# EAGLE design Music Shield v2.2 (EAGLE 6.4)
music shield
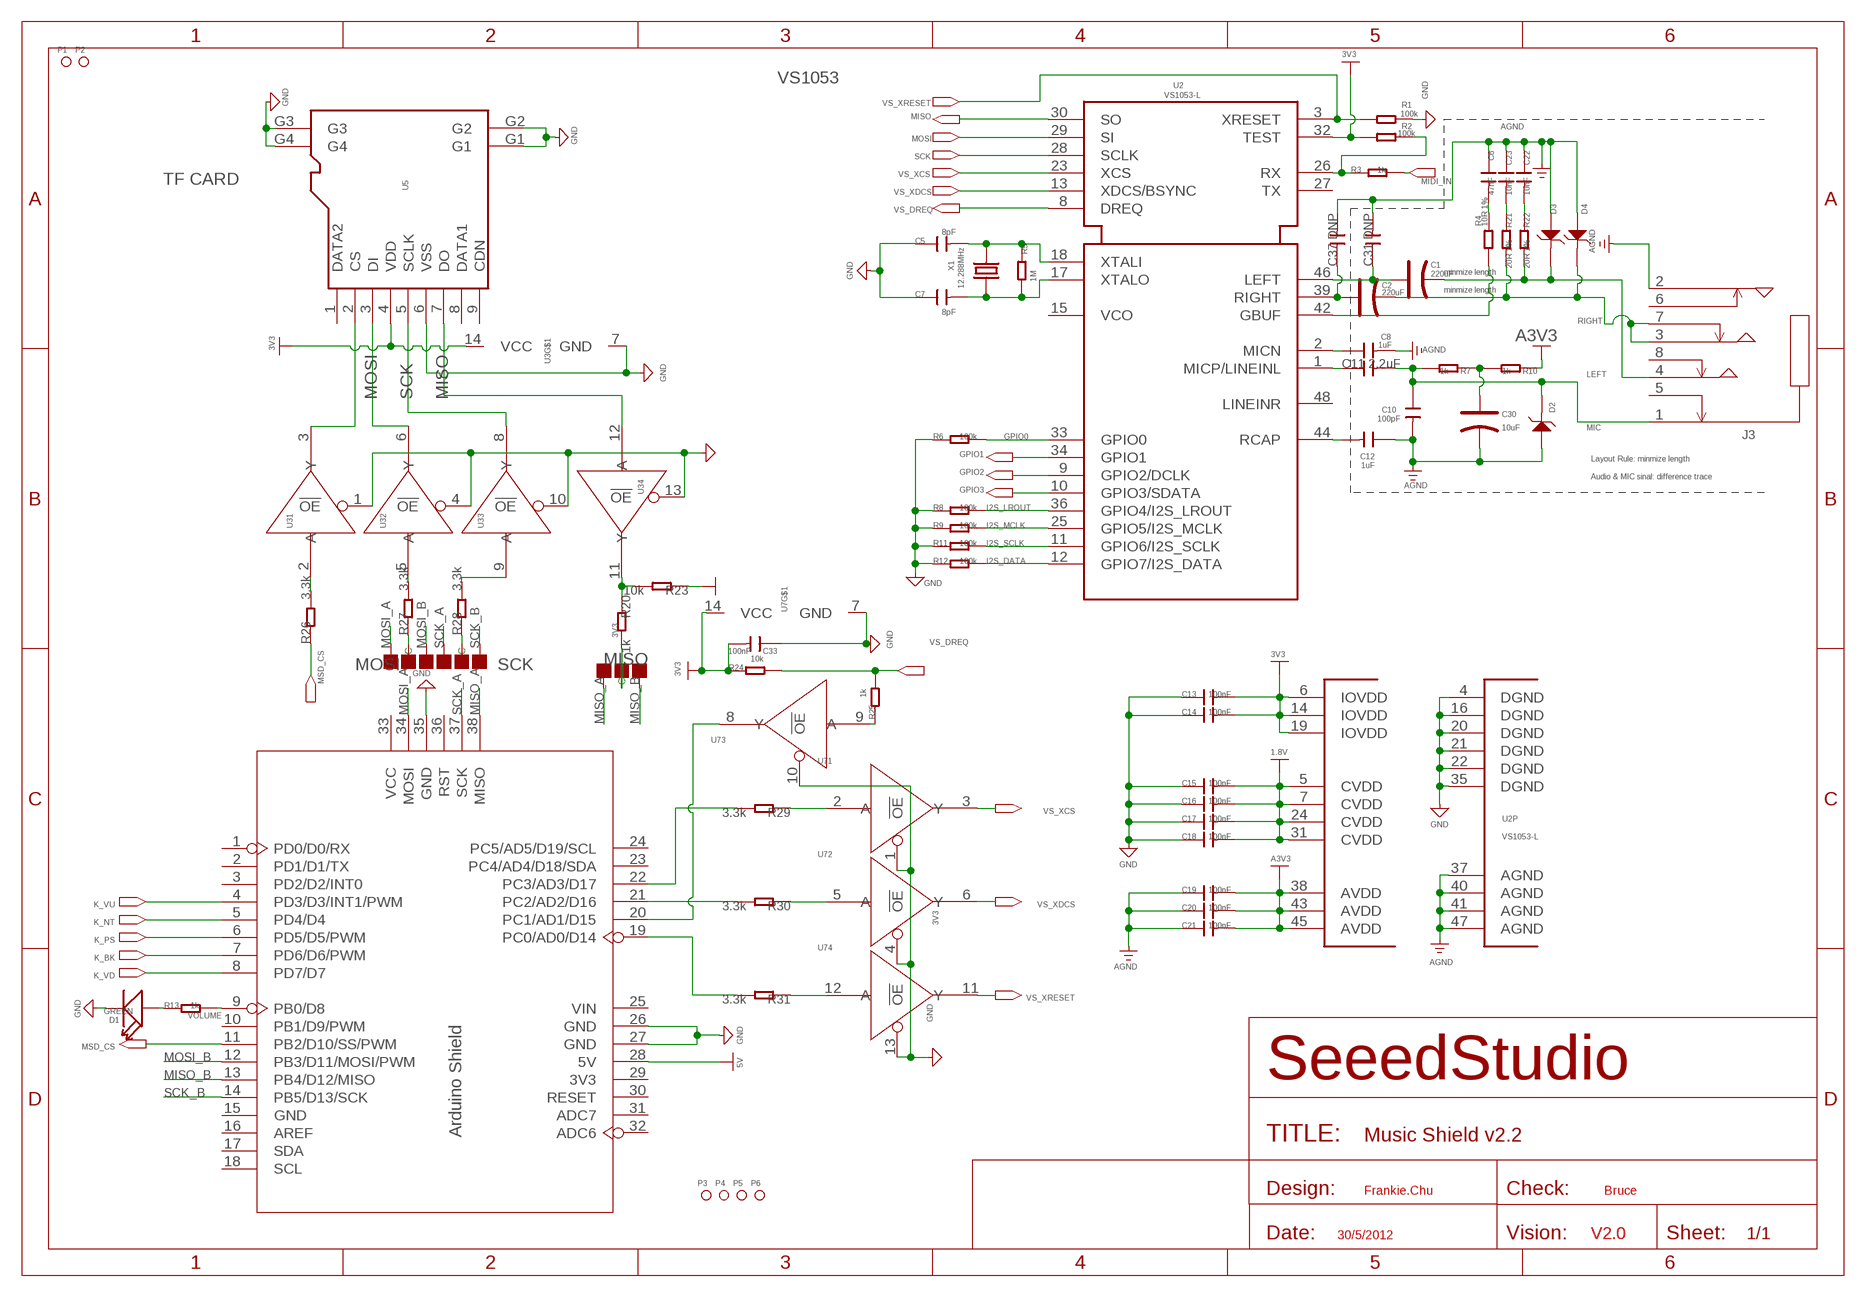
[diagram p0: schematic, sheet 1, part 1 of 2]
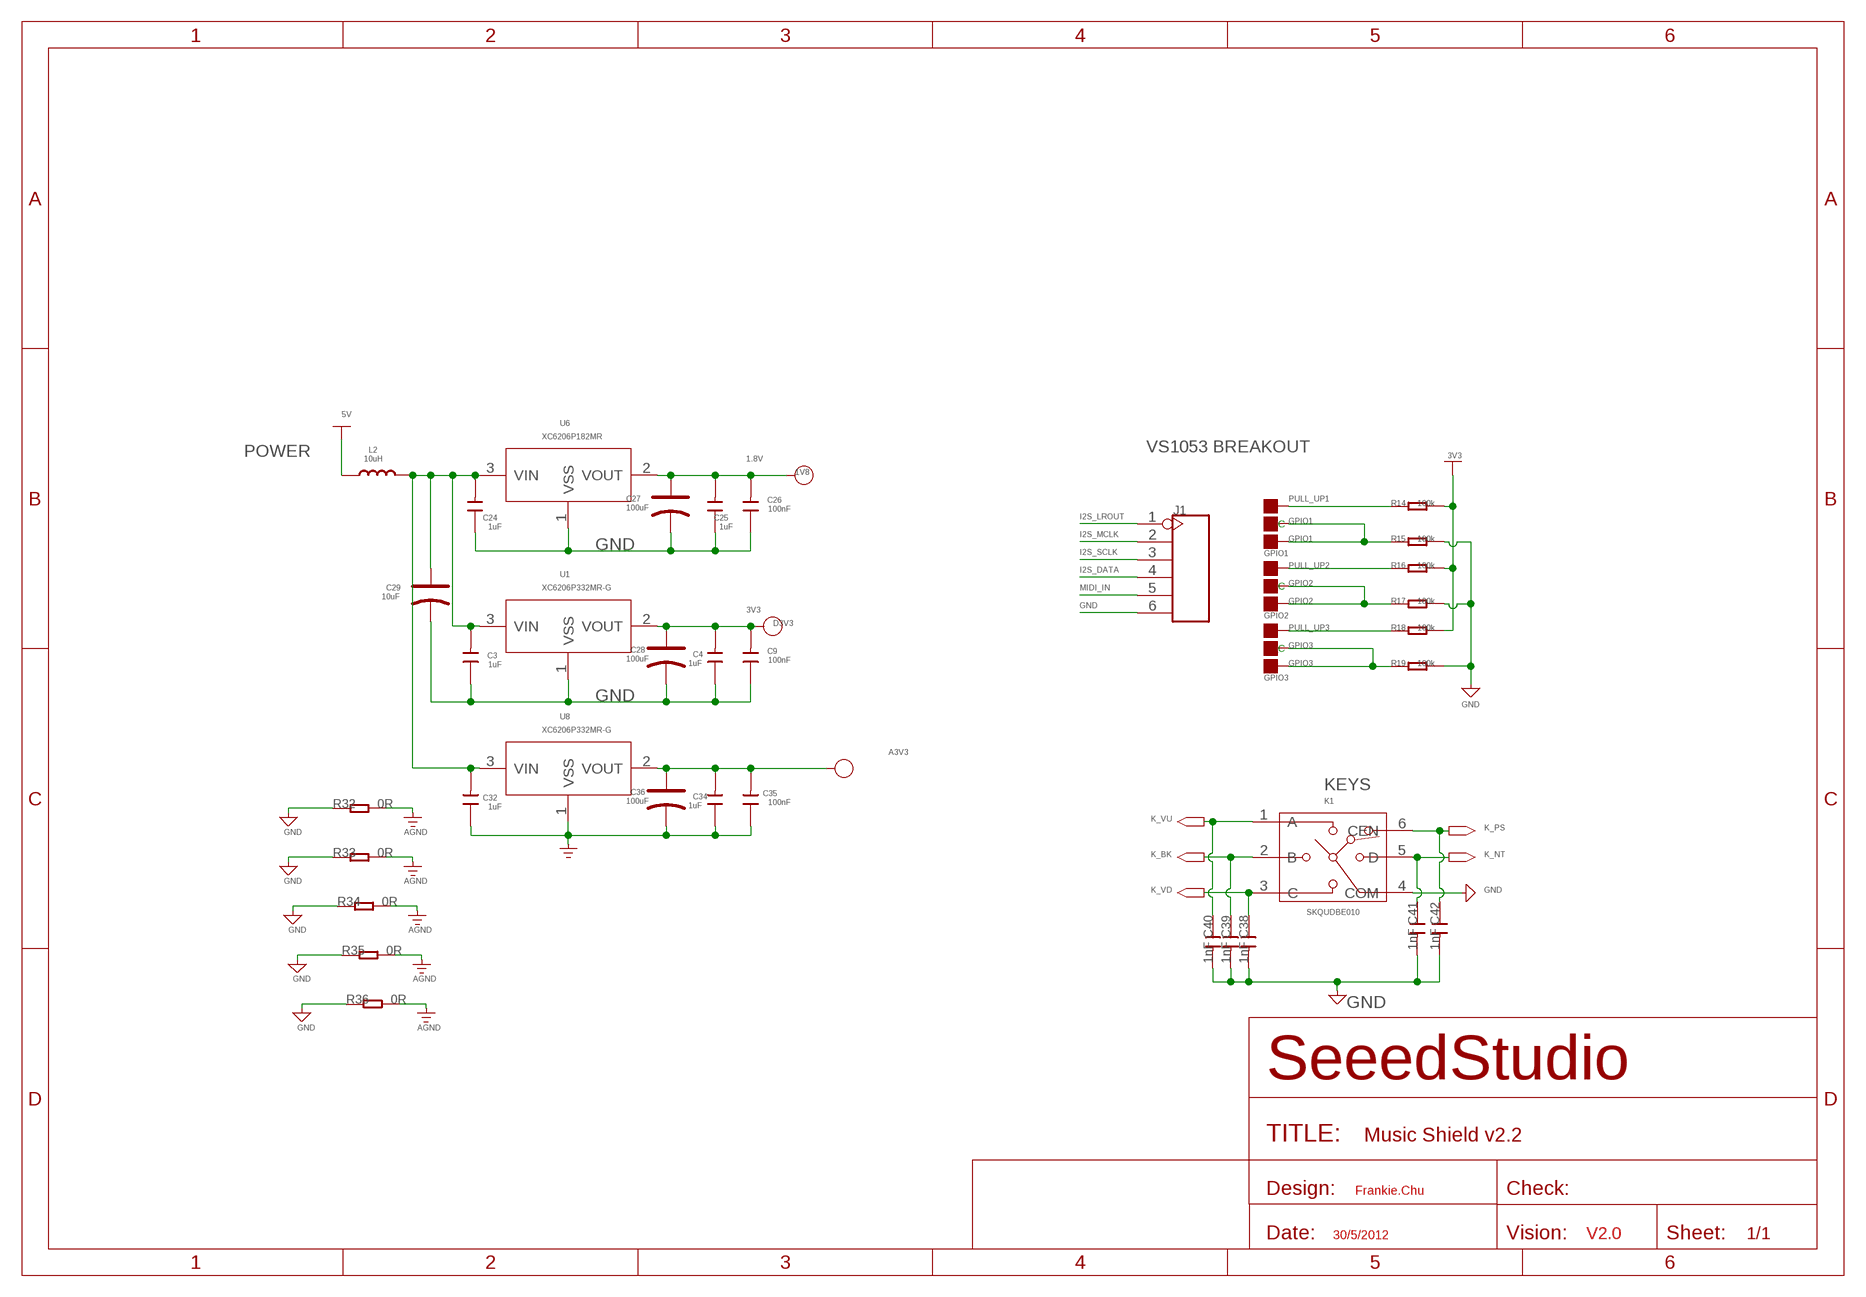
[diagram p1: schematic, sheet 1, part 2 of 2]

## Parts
1V8  PAD-TEST-POINT'4545'  [TP_4545]
A3V3  PAD-TEST-POINT'4545'  [TP_4545]
C1  220uF  CAP-AVX-B  [AVX-B]
C2  220uF  CAP-AVX-B  [AVX-B]
C3  1uF  C-0603  [C0603]
C4  1uF  C-0603  [C0603]
C5  8pF  C-0603  [C0603]
C6  47nF  C-0603  [C0603]
C7  8pF  C-0603  [C0603]
C8  1uF  C-0603  [C0603]
C9  100nF  C-0603  [C0603]
C10  100pF  C-0603  [C0603]
C11  2.2uF  C-0805  [C0805]
C12  1uF  C-0603  [C0603]
C13  100nF  C-0603  [C0603]
C14  100nF  C-0603  [C0603]
C15  100nF  C-0603  [C0603]
C16  100nF  C-0603  [C0603]
C17  100nF  C-0603  [C0603]
C18  100nF  C-0603  [C0603]
C19  100nF  C-0603  [C0603]
C20  100nF  C-0603  [C0603]
C21  100nF  C-0603  [C0603]
C22  10nF  C-0603  [C0603]
C23  10nF  C-0603  [C0603]
C24  1uF  C-0603  [C0603]
C25  1uF  C-0603  [C0603]
C26  100nF  C-0603  [C0603]
C27  100uF  CAP-AVX-B  [AVX-B]
C28  100uF  CAP-AVX-B  [AVX-B]
C29  10uF  CAP-AVX-A  [AVX-A]
C30  10uF  CAP-AVX-A  [AVX-A]
C31  DNP  C-0603  [C0603]
C32  1uF  C-0603  [C0603]
C33  100nF  C-0603  [C0603]
C34  1uF  C-0603  [C0603]
C35  100nF  C-0603  [C0603]
C36  100uF  CAP-AVX-B  [AVX-B]
C37  DNP  C-0603  [C0603]
C38  1nF  C-0603  [C0603]
C39  1nF  C-0603  [C0603]
C40  1nF  C-0603  [C0603]
C41  1nF  C-0603  [C0603]
C42  1nF  C-0603  [C0603]
D1  GREEN  LED'0603'  [LED-0603]
D2  CESD5V0D1  D-ESD  [SOD123-2.7X1.6]
D3  CESD5V0D1  D-ESD  [SOD123-2.7X1.6]
D3V3  PAD-TEST-POINT'4545'  [TP_4545]
D4  CESD5V0D1  D-ESD  [SOD123-2.7X1.6]
GPIO1  PAD-JUMPER-3P-40*40  [3P-SMD-4.1X1.5]
GPIO2  PAD-JUMPER-3P-40*40  [3P-SMD-4.1X1.5]
GPIO3  PAD-JUMPER-3P-40*40  [3P-SMD-4.1X1.5]
J1  HEADER-6P-55/35MIL  [6P-2.54-55/35MIL]
J3  AUDIO-JACK-3.5'PJ-393'  [8P-SMD-3.5]
K1  SKQUDBE010  [6P-10X10X8.6MM]
L2  10uH  L'0806'  [0806]
MISO  PAD-JUMPER-3P-40*40  [3P-SMD-4.1X1.5]
MOSI  PAD-JUMPER-3P-40*40  [3P-SMD-4.1X1.5]
P1  PAD-MARK'ANNULAR'  [ROUND-MARK-1.0]
P2  PAD-MARK'ANNULAR'  [ROUND-MARK-1.0]
P3  PAD-MARK'ANNULAR'  [ROUND-MARK-1.0]
P4  PAD-MARK'ANNULAR'  [ROUND-MARK-1.0]
P5  PAD-MARK'ANNULAR'  [ROUND-MARK-1.0]
P6  PAD-MARK'ANNULAR'  [ROUND-MARK-1.0]
R1  100k  R-0603  [R0603]
R2  100k  R-0603  [R0603]
R3  1k  R-0603  [R0603]
R4  10R 1%  R-0603  [R0603]
R5  1M  R-0603  [R0603]
R6  100k  R-0603  [R0603]
R7  1k  R-0603  [R0603]
R8  100k  R-0603  [R0603]
R9  100k  R-0603  [R0603]
R10  1k  R-0603  [R0603]
R11  100k  R-0603  [R0603]
R12  100k  R-0603  [R0603]
R13  1k  R-0603  [R0603]
R14  100k  R-0603  [R0603]
R15  100k  R-0603  [R0603]
R16  100k  R-0603  [R0603]
R17  100k  R-0603  [R0603]
R18  100k  R-0603  [R0603]
R19  100k  R-0603  [R0603]
R20  1k  R-0603  [R0603]
R21  20R 1%  R-0603  [R0603]
R22  20R 1%  R-0603  [R0603]
R23  10k  R-0603  [R0603]
R24  10k  R-0603  [R0603]
R25  1k  R-0603  [R0603]
R26  3.3k  R-0603  [R0603]
R27  3.3k  R-0603  [R0603]
R28  3.3k  R-0603  [R0603]
R29  3.3k  R-0603  [R0603]
R30  3.3k  R-0603  [R0603]
R31  3.3k  R-0603  [R0603]
R32  0R  R-0603  [R0603]
R33  0R  R-0603  [R0603]
R34  0R  R-0603  [R0603]
R35  0R  R-0603  [R0603]
R36  0R  R-0603  [R0603]
SCK  PAD-JUMPER-3P-40*40  [3P-SMD-4.1X1.5]
U1  XC6206P332MR-G  XC6206MR  [SOT23]
U2  VS1053-L  [LQFP48]
U3  74VHC125MTCX  74VHC125PW  [TSSOP14]
U5  HOLDER-MICROSD-9P'HOLDER'  [9P-SMD-W/-RING]
U6  XC6206P182MR  XC6206MR  [SOT23]
U7  74VHC125MTCX  74VHC125PW  [TSSOP14]
U8  XC6206P332MR-G  XC6206MR  [SOT23]
U10  ARDUINO-38P'WITH/O-SILK'  [ARDUINO-38P-500519002]
X1  12.288MHz  CRYSTAL'5032'  [2P-SMD-5X3.2]

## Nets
1.8V: 1V8.T C15.2 C16.2 C17.2 C18.2 C25.2 C26.2 C27.+ U2.5(CVDD) U2.7(CVDD) U2.24(CVDD) U2.31(CVDD) U6.2(VOUT) ; supply symbol labelled POWER_BAR
3V3: C4.2 C9.2 C13.2 C14.2 C28.+ C33.2 D3V3.T R2.1 R14.2 R16.2 R18.2 R23.1 R24.1 U1.2(VOUT) U2.6(IOVDD) U2.14(IOVDD) U2.19(IOVDD) U2.32(TEST) U3.14(VCC) U5.4(VDD) U7.14(VCC) ; supply symbol labelled POWER_BAR
5V: L2.1 U10.28(5V) ; supply symbol labelled POWER_BAR
A3V3: A3V3.T C19.2 C20.2 C21.2 C34.2 C35.2 C36.+ R10.1 U2.38(AVDD) U2.43(AVDD) U2.45(AVDD) U8.2(VOUT) ; supply symbol labelled POWER_BAR
AGND: C6.1 C8.2 C10.2 C12.1 C19.1 C20.1 C21.1 C22.1 C23.1 C30.- C31.2 C32.1 C34.1 C35.1 C36.- C37.2 D2.1 D3.1 D4.1 J3.2 R32.2 R33.2 R34.2 R35.2 R36.2 U2.37(AGND) U2.40(AGND) U2.41(AGND) U2.47(AGND) U8.1(VSS)
GND: C3.1 C4.1 C5.1 C7.1 C9.1 C13.1 C14.1 C15.1 C16.1 C17.1 C18.1 C24.1 C25.1 C26.1 C27.- C28.- C29.- C33.1 C38.2 C39.2 C40.2 C41.2 C42.2 D1.- J1.6 K1.4(COM) R1.2 R6.1 R8.1 R9.1 R11.1 R12.1 R15.2 R17.2 R19.2 R32.1 R33.1 R34.1 R35.1 R36.1 U1.1(VSS) U2.4(DGND) U2.16(DGND) U2.20(DGND) U2.21(DGND) U2.22(DGND) U2.35(DGND) U3.1(1:!OE) U3.4(2:!OE) U3.7(GND) U3.10(3:!OE) U3.13(4:!OE) U5.6(VSS) U5.G1 U5.G2 U5.G3 U5.G4 U6.1(VSS) U7.1(1:!OE) U7.4(2:!OE) U7.7(GND) U7.10(3:!OE) U7.13(4:!OE) U10.26(GND) U10.27(GND) U10.35(GND) ; supply symbol labelled GND_SIGNAL
GPIO0: R6.2 U2.33(GPIO0)
GPIO1: GPIO1.00(L) GPIO1.MM(C) R15.1 U2.34(GPIO1)
GPIO2: GPIO2.00(L) GPIO2.MM(C) R17.1 U2.9(GPIO2/DCLK)
GPIO3: GPIO3.00(L) GPIO3.MM(C) R19.1 U2.10(GPIO3/SDATA)
I2S_DATA: J1.4 R12.2 U2.12(GPIO7/I2S_DATA)
I2S_LROUT: J1.1 R8.2 U2.36(GPIO4/I2S_LROUT)
I2S_MCLK: J1.2 R9.2 U2.25(GPIO5/I2S_MCLK)
I2S_SCLK: J1.3 R11.2 U2.11(GPIO6/I2S_SCLK)
K_BK: C39.1 K1.2(B) U10.7(PD6/D6/PWM)
K_NT: C41.1 K1.5(D) U10.5(PD4/D4)
K_PS: C42.1 K1.6(CEN) U10.6(PD5/D5/PWM)
K_VD: C38.1 K1.3(C) U10.8(PD7/D7)
K_VU: C40.1 K1.1(A) U10.4(PD3/D3/INT1/PWM)
LEFT: C1.- D3.2 J3.4 R22.2
MIC: C10.1 C11.2 D2.2 J3.1 R7.2
MIDI_IN: J1.5 R3.2
MISO: U2.30(SO) U3.12(4:A) U5.7(DO)
MISO_A: MISO.00(L) U10.38(MISO)
MISO_B: MISO.11(R) U10.13(PB4/D12/MISO)
MOSI: U2.29(SI) U3.6(2:Y) U5.3(DI)
MOSI_A: MOSI.11(R) U10.34(MOSI)
MOSI_B: MOSI.00(L) U10.12(PB3/D11/MOSI/PWM)
MSD_CS: R26.1 U10.11(PB2/D10/SS/PWM)
N$1: C5.2 R5.1 U2.18(XTALI) X1.2
N$2: C7.2 R5.2 U2.17(XTALO) X1.1
N$3: C12.2 U2.44(RCAP)
N$4: C30.+ R7.1 R10.2
N$5: C22.2 R22.1
N$6: C2.+ C37.1 U2.39(RIGHT)
N$7: C8.1 U2.2(MICN)
N$8: C1.+ C31.1 U2.46(LEFT)
N$9: C6.2 R4.2
N$10: C23.2 R21.1
N$11: C11.1 U2.1(MICP/LINEINL)
N$12: R2.2 R3.1 U2.26(RX)
N$13: C3.2 C24.2 C29.+ C32.2 L2.2 U1.3(VIN) U6.3(VIN) U8.3(VIN)
N$14: R31.2 U10.19(PC0/AD0/D14)
N$15: R4.1 U2.42(GBUF)
N$16: R26.2 U3.2(1:A)
N$17: R29.1 U7.2(1:A)
N$18: R27.2 U3.5(2:A)
N$19: R30.1 U7.5(2:A)
N$20: R31.1 U7.12(4:A)
N$21: U3.3(1:Y) U5.2(CS)
N$22: R29.2 U10.22(PC3/AD3/D17)
N$23: R30.2 U10.21(PC2/AD2/D16)
N$24: U7.8(3:Y) U10.20(PC1/AD1/D15)
N$36: R20.1 R23.2 U3.11(4:Y)
N$37: D1.+ R13.1
N$38: R25.1 U7.9(3:A)
N$39: MISO.MM(C) R20.2
N$40: R28.2 U3.9(3:A)
N$49: MOSI.MM(C) R27.1
N$53: R28.1 SCK.MM(C)
PULL_UP1: GPIO1.11(R) R14.1
PULL_UP2: GPIO2.11(R) R16.1
PULL_UP3: GPIO3.11(R) R18.1
RIGHT: C2.- D4.2 J3.3 J3.7 R21.2
SCK: U2.28(SCLK) U3.8(3:Y) U5.5(SCLK)
SCK_A: SCK.11(R) U10.37(SCK)
SCK_B: SCK.00(L) U10.14(PB5/D13/SCK)
VOLUME: R13.2 U10.9(PB0/D8)
VS_DREQ: R24.2 R25.2 U2.8(DREQ)
VS_XCS: U2.23(XCS) U7.3(1:Y)
VS_XDCS: U2.13(XDCS/BSYNC) U7.6(2:Y)
VS_XRESET: R1.1 U2.3(XRESET) U7.11(4:Y)
Unconnected: J3.5 J3.6 J3.8 U2.15(VCO) U2.27(TX) U2.48(LINEINR) U5.1(DATA2) U5.8(DATA1) U5.9(CDN) U10.1(PD0/D0/RX) U10.2(PD1/D1/TX) U10.3(PD2/D2/INT0) U10.10(PB1/D9/PWM) U10.15(GND) U10.16(AREF) U10.17(SDA) U10.18(SCL) U10.23(PC4/AD4/D18/SDA) U10.24(PC5/AD5/D19/SCL) U10.25(VIN) U10.29(3V3) U10.30(RESET) U10.31(ADC7) U10.32(ADC6) U10.33(VCC) U10.36(RST)

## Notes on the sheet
- VS1053
- TF CARD
- minmize length
- minmize length
- POWER | VS1053 BREAKOUT
- Layout Rule: minmize length
- Audio & MIC sinal: difference trace
- KEYS
- Arduino Shield
- Frankie.Chu | Bruce | Frankie.Chu
- 30/5/2012 | V2.0 | 30/5/2012 | V2.0

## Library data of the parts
1V8 A3V3 D3V3 = Discrete:PAD-TEST-POINT; PARTNO: DNP
C1 C2 C27-C30 C36 = Discrete:CAP*: Electrolytic Capacitors,Tantalum Capacitors and Super Capacitors
C3-C26 C31-C35 C37-C42 = Discrete:C*: Ceramic Capacitors
D1 = Discrete:LED*
D2-D4 = template:D-ESD: Diodes for Protectiong against ESD
GPIO1-GPIO3 MISO MOSI SCK = Discrete:PAD-JUMPER-3P; PARTNO: DNP
J1 = Connector:HEADER-6P
J3 = template:AUDIO-JACK-3.5
K1 = template:SKQUDBE010: four dircction and center button
L2 = Discrete:L*
P1-P6 = Discrete:PAD-MARK; PARTNO: DNP
R1-R36 = Discrete:R*
U1 U6 U8 = IC:XC6206: LOW ESR Cap.Compatible Positive Voltage Regulators
U2 = vlsi:VS1053
U3 U7 = template:74V*125: Quad Buffer/Line Driver;3-state
U5 = Connector:HOLDER-MICROSD-9P
U10 = moudle:ARDUINO-38P
X1 = Discrete:CRYSTAL*: CRYSTAL

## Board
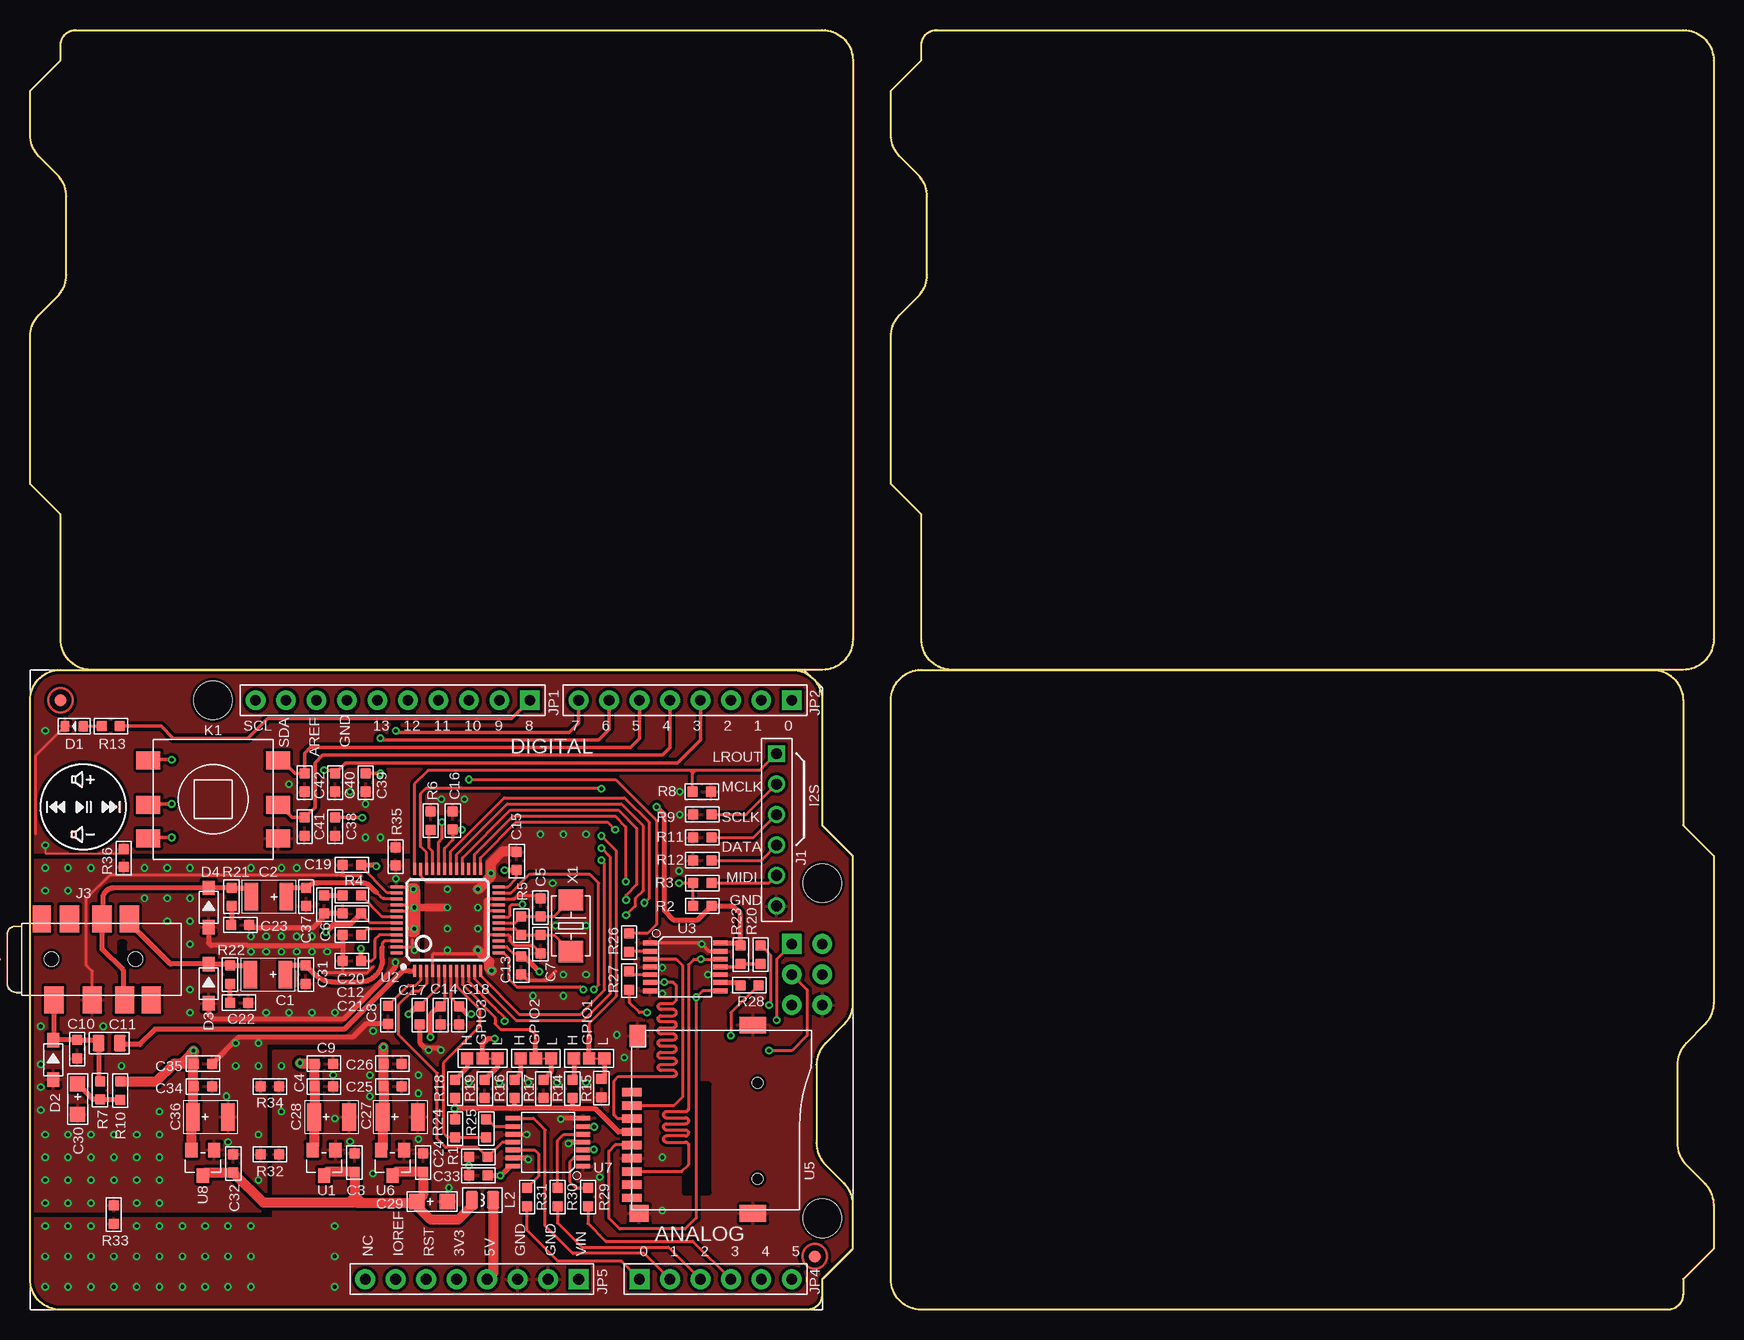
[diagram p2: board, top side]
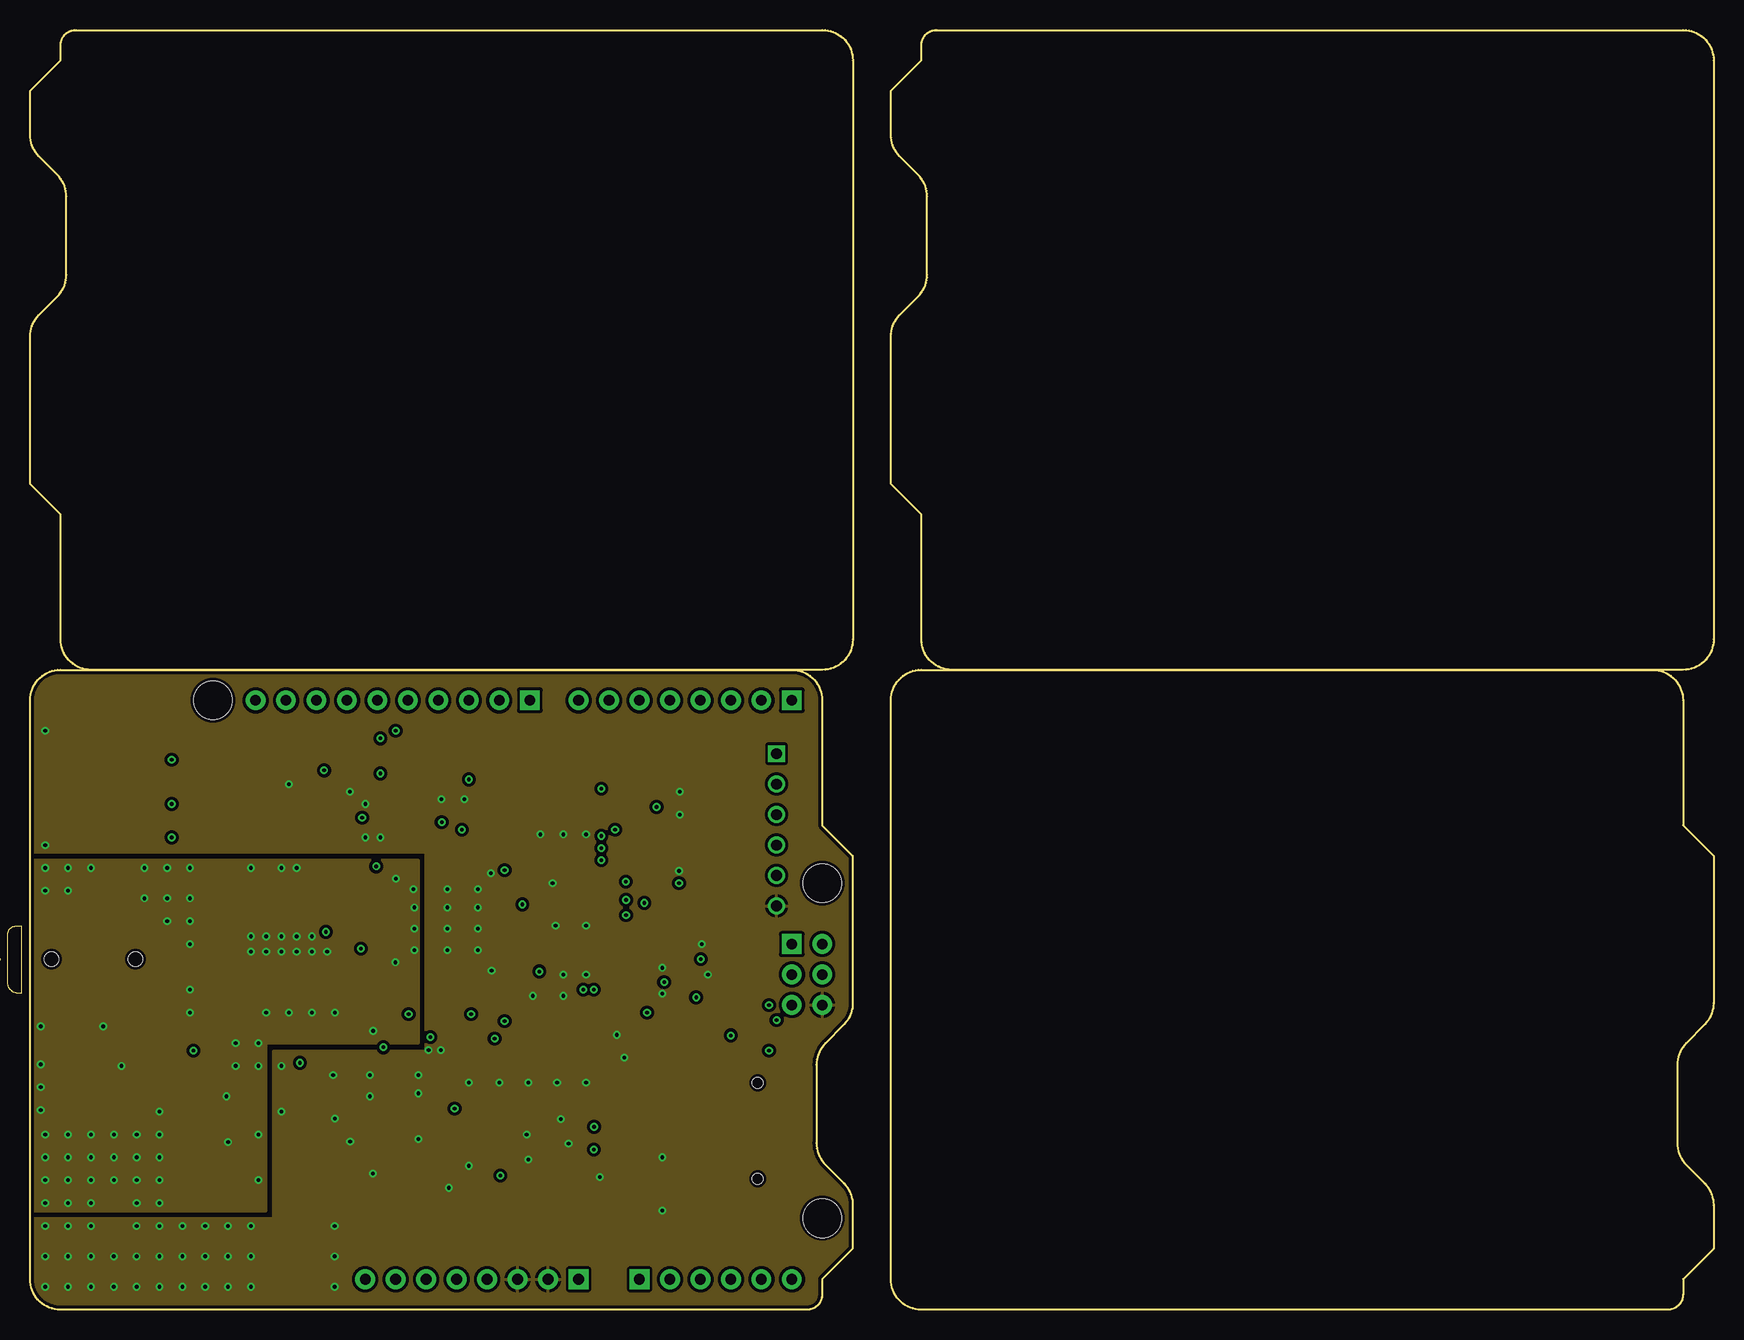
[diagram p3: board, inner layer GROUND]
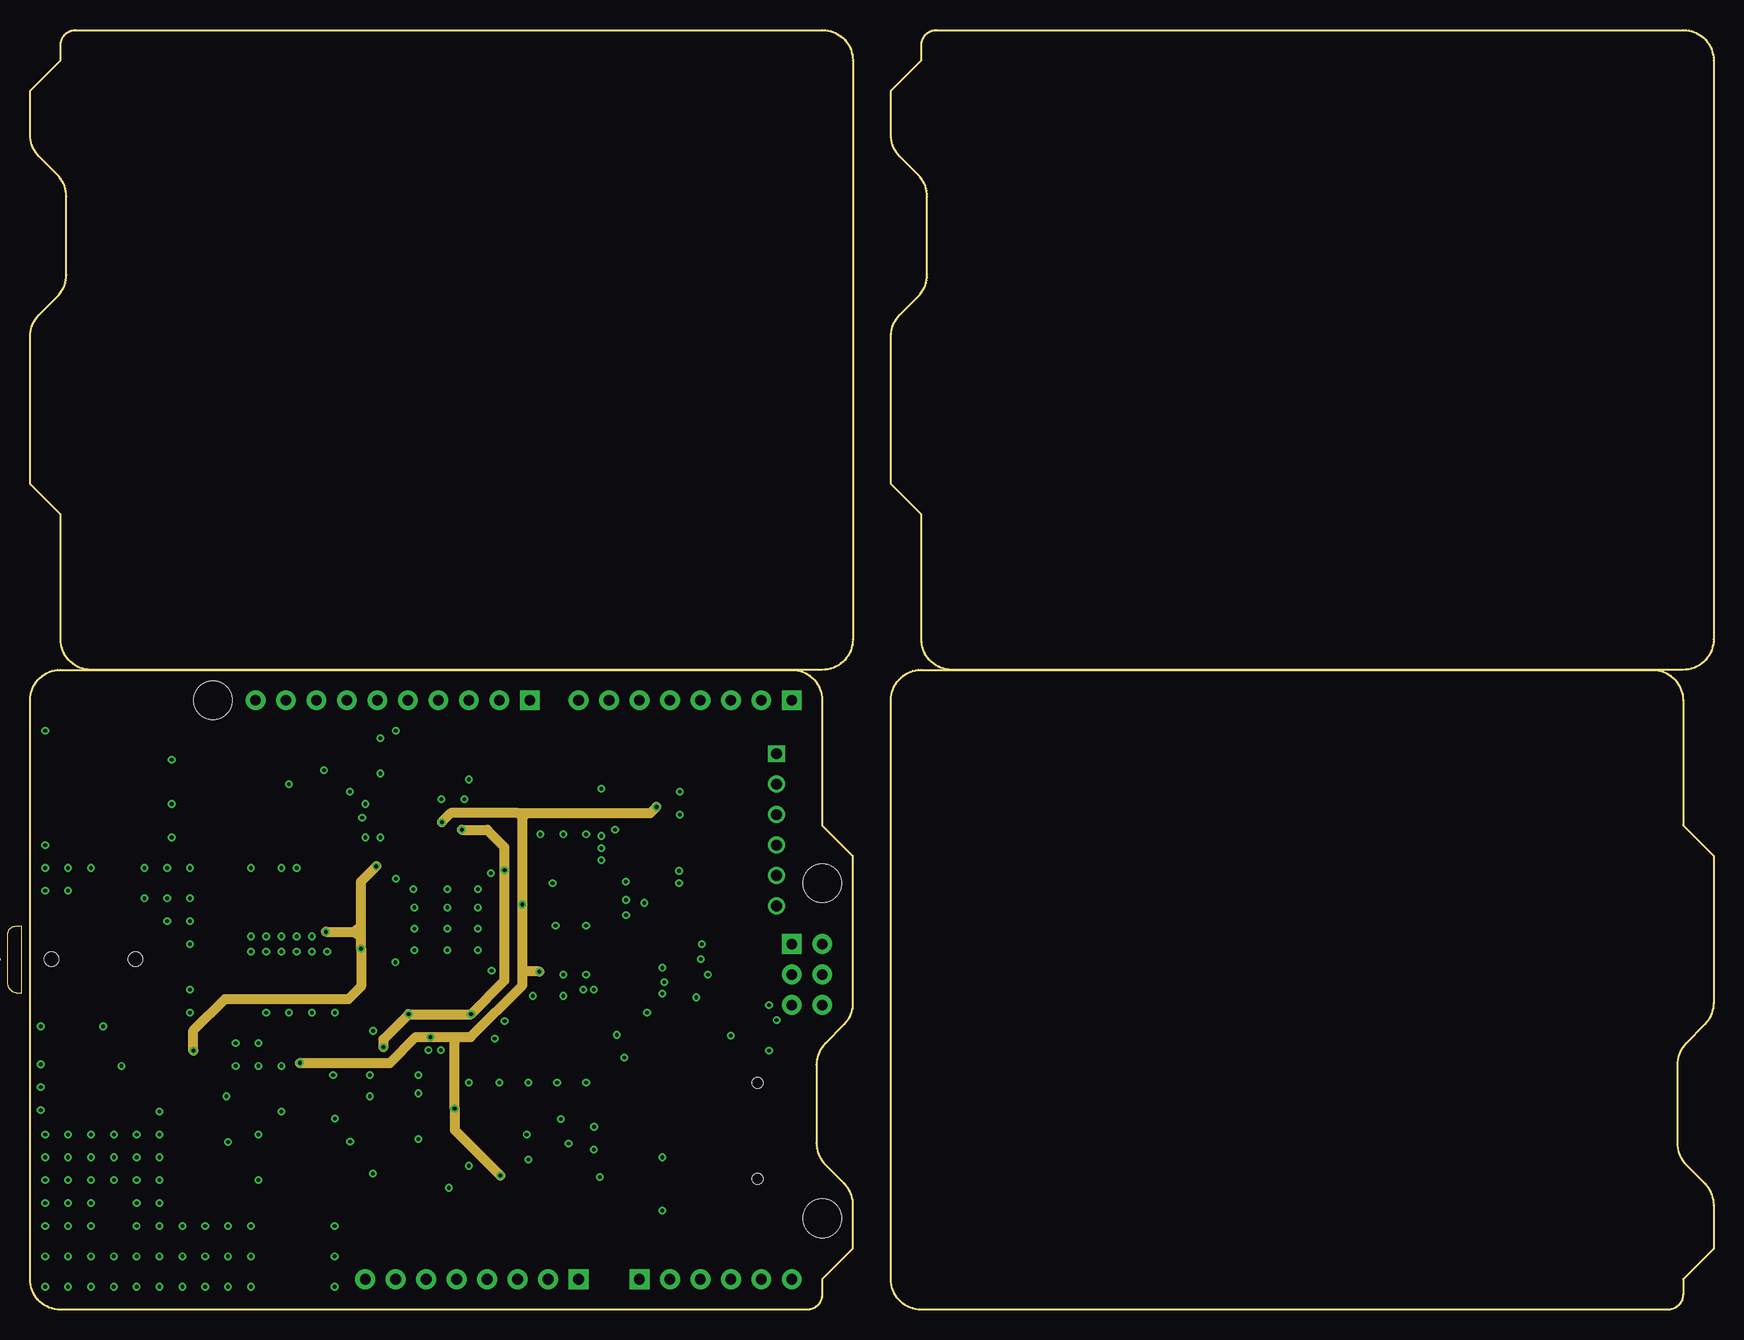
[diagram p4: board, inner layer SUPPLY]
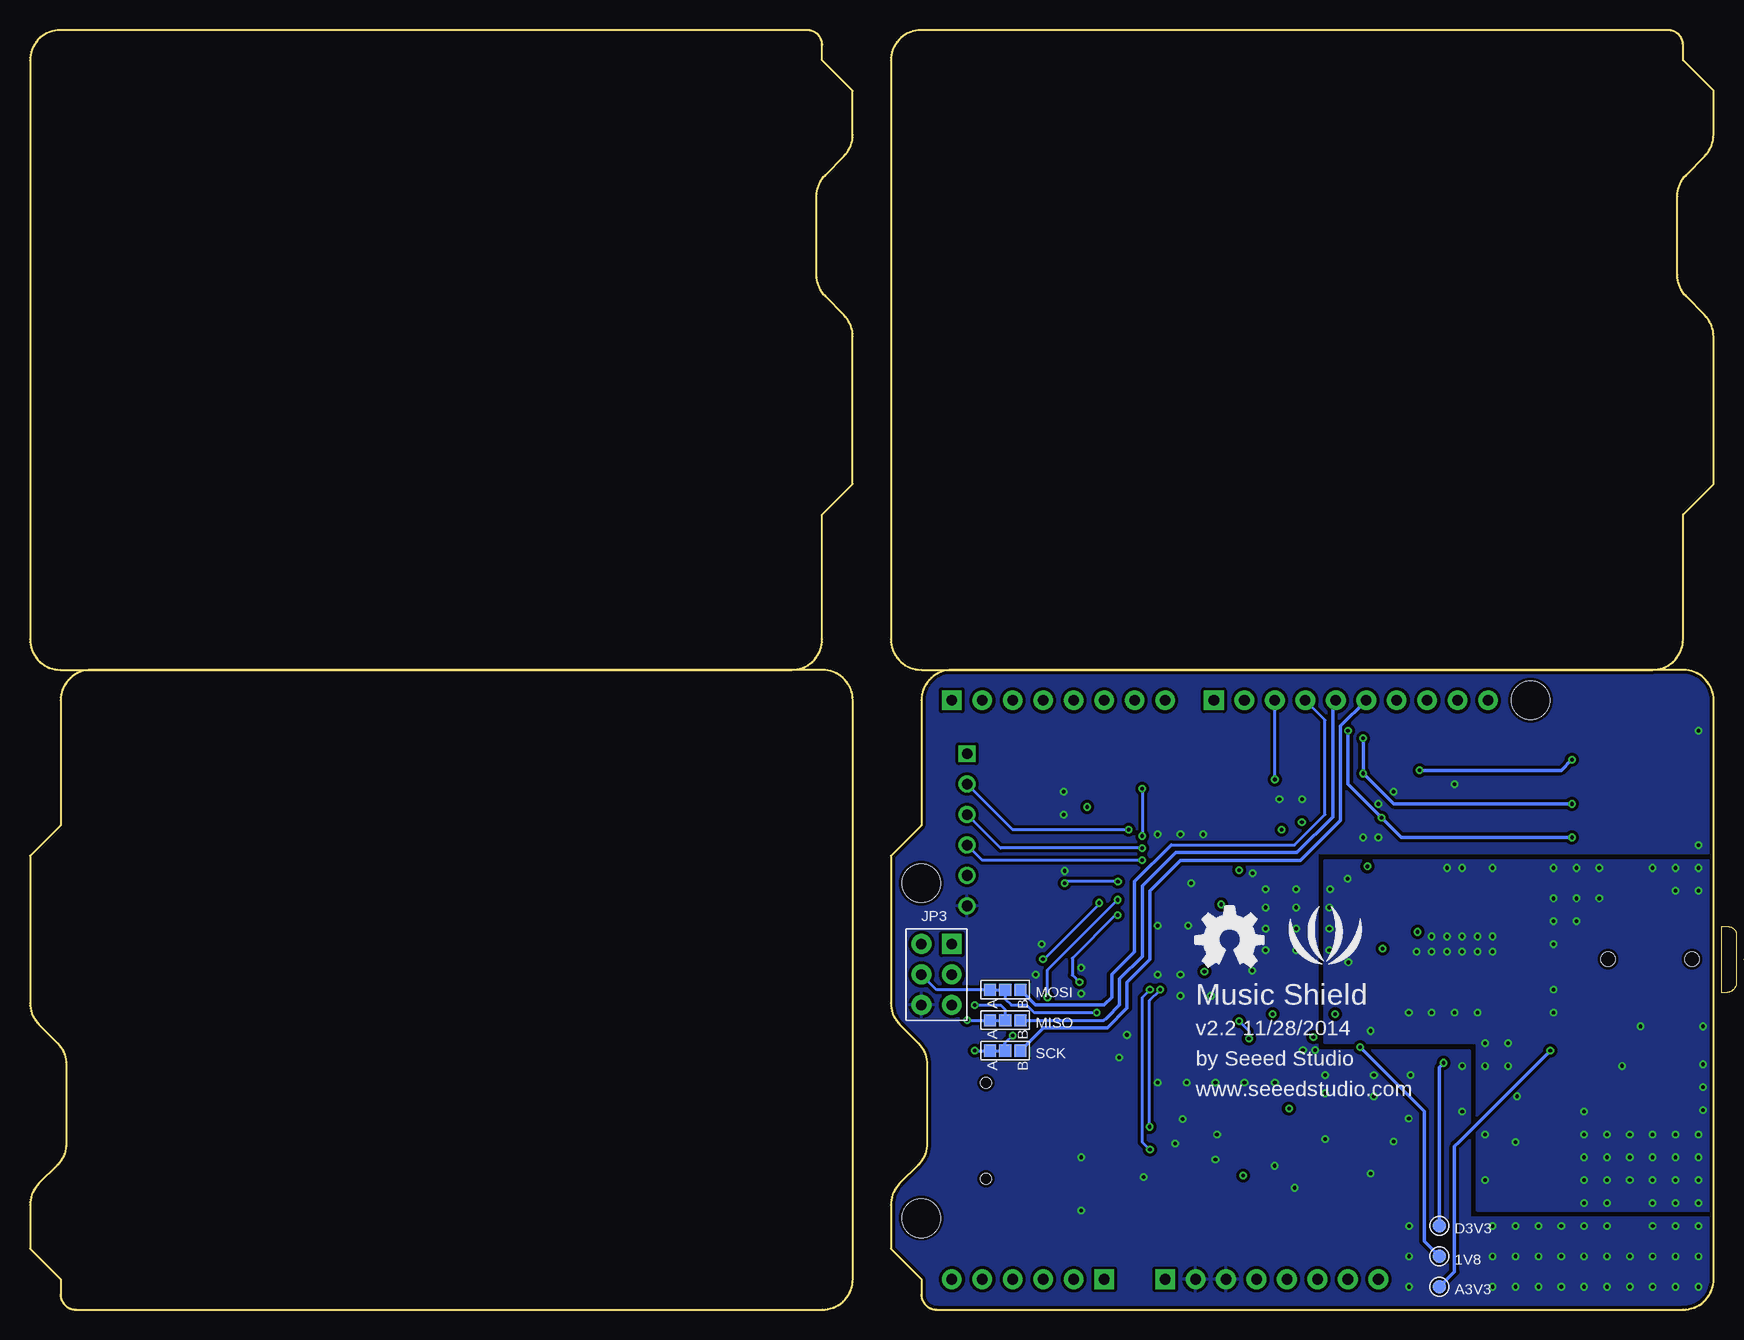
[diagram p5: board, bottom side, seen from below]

Size 140.34 x 106.68 mm. Coordinates in mm from the lower left corner, seen from the top.
Outline: 80 segments
Copper layers (1*16): Top 0.035mm / dielectric 1.5mm / Bottom 0.035mm
Design rules "SeeedStudio_2layer_DRU_no_angle_20140221 *": minimum track width 6mil, minimum drill 12mil, track to track 6mil, track to pad 6mil, pad to pad 6mil, via to via 6mil, smd to smd 0mil, copper to edge 10mil, drill to drill 10mil, minimum pad ring 10mil, minimum via ring 6mil, stop-mask expansion 2mil, vias tented up to drill 100mil, thermal gap 10mil
Holes 2.03 mm at 7.62,111.12 132.72,111.12 132.72,-4.45 7.62,-4.45
tRestrict: area 26.6,33.3 to 27.1,33.5; area 30.2,33.5 to 30.7,33.6; area 7.5,28.1 to 7.9,30.6; area 38.7,34 to 39.2,34.1; area 38.7,33.5 to 39.2,33.6

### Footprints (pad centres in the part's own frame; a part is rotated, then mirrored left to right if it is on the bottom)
TP_4545 = smd 1.143 x 1.143: T 0,0
AVX-B = smd 1.143 x 2.286: + -1.46,0; - 1.46,0
C0603 = smd 0.889 x 0.889: 1 -0.762,0; 2 0.762,0
C0805 = smd 1.016 x 1.397: 1 -0.889,0; 2 0.889,0
AVX-A = smd 1.27 x 1.27: + -1.27,0; - 1.27,0
LED-0603 = smd 0.762 x 0.889: + -0.762,0; - 0.762,0
SOD123-2.7X1.6 = smd 1.2 x 1.02: 1 -1.635,0; 2 1.635,0
3P-SMD-4.1X1.5 = smd 1.016 x 1.016: 00 -1.27,0; 11 1.27,0; MM 0,0
6P-2.54-55/35MIL = drill 0.889 pad 1.397 square: 1 0,6.35 | drill 0.889 pad 1.397: 2 0,3.81; 3 0,1.27; 4 0,-1.27; 5 0,-3.81; 6 0,-6.35
8P-SMD-3.5 = smd 1.6 x 2.25: 1 3.9,-3.375; 2 7.1,-3.375; 3 9.8,-3.375; 4 10.2,3.375; 6 5.2,3.375; 7 7.9,3.375; 8 12,-3.375 | smd 1.5 x 2.25: 5 2.9,3.375 | hole 1.2: 3.7,0; 10.7,0
6P-10X10X8.6MM = smd 2 x 1.5: 1 -5.4,3.25; 2 -5.4,-0.45; 3 -5.4,-3.25; 4 5.4,-3.25; 5 5.4,-0.45; 6 5.4,3.25
0806 = smd 1.016 x 1.524: 1 -0.889,0; 2 0.889,0
ROUND-MARK-1.0 = smd 1.016 x 1.016: P$1 0,0
R0603 = smd 0.889 x 0.889: 1 -0.762,0; 2 0.762,0
SOT23 = smd 1.016 x 1.2: 1 -0.95,-1.06; 2 0.95,-1.06; 3 0,1.06
LQFP48 = smd 0.25 x 1: 1 -2.75,-4.25; 2 -2.25,-4.25; 3 -1.75,-4.25; 4 -1.25,-4.25; 5 -0.75,-4.25; 6 -0.25,-4.25; 7 0.25,-4.25; 8 0.75,-4.25; 9 1.25,-4.25; 10 1.75,-4.25; 11 2.25,-4.25; 12 2.75,-4.25; 25 2.75,4.25; 26 2.25,4.25; 27 1.75,4.25; 28 1.25,4.25; 29 0.75,4.25; 30 0.25,4.25; 31 -0.25,4.25; 32 -0.75,4.25; 33 -1.25,4.25; 34 -1.75,4.25; 35 -2.25,4.25; 36 -2.75,4.25 | smd 1 x 0.25: 13 4.25,-2.75; 14 4.25,-2.25; 15 4.25,-1.75; 16 4.25,-1.25; 17 4.25,-0.75; 18 4.25,-0.25; 19 4.25,0.25; 20 4.25,0.75; 21 4.25,1.25; 22 4.25,1.75; 23 4.25,2.25; 24 4.25,2.75; 37 -4.25,2.75; 38 -4.25,2.25; 39 -4.25,1.75; 40 -4.25,1.25; 41 -4.25,0.75; 42 -4.25,0.25; 43 -4.25,-0.25; 44 -4.25,-0.75; 45 -4.25,-1.25; 46 -4.25,-1.75; 47 -4.25,-2.25; 48 -4.25,-2.75
TSSOP14 = smd 0.4 x 1.2: 1 -2,-2.925; 2 -1.3,-2.925; 3 -0.65,-2.925; 4 0,-2.925; 5 0.65,-2.925; 6 1.3,-2.925; 7 2,-2.925; 8 2,2.925; 9 1.3,2.925; 10 0.65,2.925; 11 0,2.925; 12 -0.65,2.925; 13 -1.3,2.925; 14 -2,2.925
9P-SMD-W/-RING = smd 1.6 x 0.7: 1 0,2.25; 2 0,1.15; 3 0,0.05; 4 0,-1.05; 5 0,-2.15; 6 0,-3.25; 7 0,-4.35; 8 0,-5.45; 9 0,-6.55 | smd 1.6 x 1.4: G1 0.6,-7.85 | smd 2.2 x 1.4: G2 10.1,-7.85; G3 10.1,7.85 | smd 1.4 x 1.8: G4 0.5,6.95 | hole 0.9: 10.5,-4.95; 10.5,3.05
ARDUINO-38P-500519002 = drill 0.889 pad 1.651 square: 1 63.5,50.8; 9 41.656,50.8; 19 50.8,2.54; 25 45.72,2.54; 38 63.5,30.48 | drill 0.889 pad 1.651: 2 60.96,50.8; 3 58.42,50.8; 4 55.88,50.8; 5 53.34,50.8; 6 50.8,50.8; 7 48.26,50.8; 8 45.72,50.8; 10 39.116,50.8; 11 36.576,50.8; 12 34.036,50.8; 13 31.496,50.8; 14 28.956,50.8; 15 26.416,50.8; 16 23.876,50.8; 17 21.336,50.8; 18 18.796,50.8; 20 53.34,2.54; 21 55.88,2.54; 22 58.42,2.54; 23 60.96,2.54; 24 63.5,2.54; 26 43.18,2.54; 27 40.64,2.54; 28 38.1,2.54; 29 35.56,2.54; 30 33.02,2.54; 31 30.48,2.54; 32 27.94,2.54; 33 66.04,30.48; 34 66.04,27.94; 35 66.04,25.4; 36 63.5,25.4; 37 63.5,27.94 | hole 3.2: 15.24,50.8; 66.04,35.56; 66.04,7.62
2P-SMD-5X3.2 = smd 1.778 x 2.032: 1 -2.159,0; 2 2.159,0

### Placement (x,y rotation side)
1V8  22.86,4.45 0 bottom
A3V3  22.86,1.91 90 bottom
C1  19.84,27.94 180 top
C2  19.93,34.42 180 top
C3  27.05,12.26 270 top
C4  24.51,18.61 180 top
C5  42.55,33.53 270 top
C6  24.54,33.78 90 top
C7  42.55,30.48 90 top
C8  29.84,24.57 270 top
C9  24.51,20.51 180 top
C10  3.94,21.72 270 top
C11  6.6,22.23 180 top
C12  26.83,31.24 0 top
C13  40.96,28.7 90 top
C14  34.23,24.54 90 top
C15  40.58,37.4 270 top
C16  35.24,40.78 270 top
C17  32.49,24.54 90 top
C18  35.78,24.54 90 top
C19  26.83,37.08 0 top
C20  26.83,33.02 0 top
C21  26.83,29.08 0 top
C22  17.43,25.59 180 top
C23  17.52,32.07 180 top
C24  32.77,12.26 270 top
C25  30.23,18.61 180 top
C26  30.23,20.51 180 top
C27  30.86,16.07 0 top
C28  25.15,16.07 0 top
C29  33.53,9.02 0 top
C30  3.97,17.56 270 top
C31  23,27.94 270 top
C32  16.95,12.19 270 top
C33  37.37,11.21 0 top
C34  14.41,18.61 180 top
C35  14.41,20.51 180 top
C36  15.05,16.07 0 top
C37  23.02,34.42 270 top
C38  25.43,40.26 270 top
C39  27.97,43.94 270 top
C40  25.43,43.94 270 top
C41  22.89,40.26 270 top
C42  22.89,43.94 270 top
D1  3.68,48.64 180 top
D2  1.94,20.83 90 top
D3  14.89,27.18 90 top
D3V3  22.86,6.99 0 bottom
D4  14.89,33.53 90 top
GPIO1  46.61,20.95 180 top
GPIO2  42.16,20.95 180 top
GPIO3  37.72,20.95 180 top
J1  62.23,40.01 0 top
J3  -1.9,29.21 0 top
K1  15.27,42.55 0 top
L2  37.72,9.14 180 top
MISO  59.06,24.13 0 bottom
MOSI  59.06,26.67 180 bottom
P1  2.54,50.8 0 top
P2  65.41,4.45 0 top
P3  not placed on the board
P4  not placed on the board
P5  not placed on the board
P6  not placed on the board
R1  37.37,12.73 180 top
R2  56.04,33.66 180 top
R3  56.04,35.56 0 top
R4  26.83,34.54 180 top
R5  40.96,32 270 top
R6  33.4,40.77 270 top
R7  5.84,18.29 90 top
R8  56.01,43.18 180 top
R9  56.04,41.27 0 top
R10  7.52,18.26 270 top
R11  56.04,39.37 0 top
R12  56.04,37.47 0 top
R13  6.73,48.64 0 top
R14  45.21,18.41 270 top
R15  47.62,18.48 270 top
R16  40.39,18.41 270 top
R17  42.8,18.41 270 top
R18  35.43,18.41 270 top
R19  37.91,18.41 270 top
R20  60.89,29.59 90 top
R21  16.79,34.42 90 top
R22  16.67,27.94 90 top
R23  59.24,29.59 270 top
R24  35.43,15.11 270 top
R25  38.03,15.11 270 top
R26  49.94,30.61 270 top
R27  49.94,27.43 90 top
R28  59.97,27.05 180 top
R29  46.51,9.4 270 top
R30  43.97,9.4 270 top
R31  41.43,9.4 270 top
R32  20.01,12.95 180 top
R33  6.99,7.94 90 top
R34  20.01,18.61 180 top
R35  30.48,37.78 270 top
R36  7.82,37.66 270 top
SCK  59.06,21.59 180 bottom
U1  24.51,12.26 180 top
U2  34.8,32.51 0 top
U3  54.61,28.57 270 top
U5  50.16,15.88 0 top
U6  30.23,12.26 180 top
U7  43.18,13.97 90 top
U8  14.41,12.26 180 top
U10  0,0 0 top
U$1  [LOGO_SILK]  32.39,30.48 0 bottom
U$2  [OSHW_FILLX200_NOTEXT]  43.18,28.57 0 bottom
X1  45.09,32 90 top

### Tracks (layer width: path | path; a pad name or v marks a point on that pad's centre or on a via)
1.8V  (via drill 0.3 pad 0.64)
  Top 0.254: U2.24 39.84,35.26 40.58,35.99 C15.2 | 32.67,25.4 32.57,25.3 C17.2 32.54,25.35 32.54,25.4 34.05,26.91 U2.5 | U2.7 35.05,26.03 C18.2 | U2.31 34.55,38.45 35.24,39.15 C16.2
  Top 0.406: v39.56,36.64 C15.2 | v31.56,24.64 32.22,25.3 C17.2 | v36.77,24.64 36.48,24.64 35.82,25.3 C18.2 | C16.2 35.99,40.02 v36,40.01
  Top 0.813: v29.46,21.87 C26.2 C25.2 29.46,16.13 C27.+ 29.4,13.44 U6.2
  SUPPLY 0.813: v29.46,21.87 29.46,22.54 v31.56,24.64 v36.77,24.64 39.56,27.43 v39.56,36.64 39.56,38.55 38.1,40.01 v36,40.01
  Bottom 0.305: 1V8.T 24.13,5.71 24.13,16.55 v29.46,21.87
3V3  (via drill 0.3 pad 0.64)
  Top 0.254: U2.14 39.74,30.26 40.29,29.72 40.7,29.72 C13.2 | U2.32 34.05,38.97 34.32,39.24 v34.32,40.64 | U2.19 39.9,32.76 40.03,32.89 40.03,33.66 40.16,33.78 v41.05,33.78 | U2.6 34.55,25.62 C14.2
  Top 0.305: 40.39,16.79 40.39,17.02 | 40.39,17.02 40.39,17.08 40.39,17.02 | 40.39,17.02 40.14,16.76 | 40.39,17.02 | 40.39,17.02 40.64,16.76
  Top 0.406: C14.2 34.09,25.3 33.37,24.57 v33.37,22.73 | 38.29,11.21 C33.2 38.16,11.18 v39.21,11.18 40,11.97 U7.14 | R18.2 35.43,16.89 | 35.43,16.8 R24.1 | C13.2 41.18,29.46 v42.45,28.19 | U3.14 58.99,30.57 59.21,30.35 | R23.1 59.21,30.35 | 59.21,30.35 59.21,33.02 58.58,33.66 R2.1 55.66,32.51 53.62,32.51 52.86,33.27 52.86,41.27 v52.23,41.91 | 45.24,16.76 45.03,16.76 | 45.03,16.76 40.64,16.76 40.42,16.76 | 40.42,16.76 40.14,16.76 35.56,16.76 35.43,16.89 | R16.2 40.39,17.08 40.39,16.79 40.42,16.76 | 45.41,16.76 45.24,16.76 | R14.2 45.21,17.14 | 45.24,16.76 45.21,16.79 45.21,17.08 | 35.43,16.89 35.43,16.8 | 35.43,16.8 v35.4,16.76 | 45.21,17.08 45.21,17.14 | 45.21,17.14 45.22,17.14 45.22,17.08 | 45.22,16.95 45.03,16.76 | 45.21,17.08 45.22,17.08 | 45.22,17.08 45.22,16.95 | 45.22,16.95 45.41,16.76 | 45.41,16.76 47.12,16.76 49.06,14.82 U5.4
  Top 0.813: U1.2 23.56,13.43 23.52,13.46 23.69,13.62 C28.+ 23.75,16.13 C4.2 23.75,20.29 23.78,20.32 23.78,20.51 C9.2 22.57,20.51 v22.51,20.57
  SUPPLY 0.813: v22.51,20.57 30,20.57 32.16,22.73 v33.37,22.73 35.08,22.73 | 35.08,22.73 35.46,22.73 | 35.46,22.73 35.72,22.73 | 35.72,22.73 36.73,22.73 41.05,27.05 41.05,28.45 | 41.05,28.45 v41.05,33.78 41.05,41.4 | v42.45,28.19 41.3,28.19 41.05,28.45 | 40.67,41.4 41.05,41.4 | 41.05,41.4 41.43,41.4 | 41.43,41.4 51.72,41.4 v52.23,41.91 | 35.46,22.73 35.4,22.67 v35.4,16.76 35.4,14.99 v39.21,11.18 | 40.67,41.4 41.05,41.02 41.43,41.4 | 35.08,22.73 35.4,22.42 35.72,22.73 | 40.67,41.4 35.08,41.4 v34.32,40.64
  Bottom 0.305: D3V3.T 22.86,20.22 v22.51,20.57
5V
  Top 0.813: L2.1 38.61,3.04 U10.28
A3V3  (via drill 0.3 pad 0.64)
  Top 0.254: U2.38 29.78,34.76 27.59,36.96 C19.2 | U2.43 28.35,32.26 C20.2 | U2.45 29.13,31.26 28.73,30.86 28.73,29.34 28.48,29.08 C21.2
  Top 0.406: C20.2 26.7,32.13 25.3,32.13 v24.67,31.5 | C21.2 v27.59,30.1 | R10.1 7.62,19.02 | C19.2 28.64,37.08 28.77,36.96 v28.86,36.96
  Top 0.813: U8.2 13.46,15.88 | 13.46,15.88 13.46,15.97 13.62,16.13 13.62,18.57 | C36.+ 13.59,16 13.46,15.88 | 13.62,18.57 C34.2 | 13.62,18.57 13.62,20.57 13.65,20.54 C35.2 | C35.2 13.65,21.52 | 7.62,19.02 10.52,19.02 12.01,20.51 C35.2 | 13.65,21.56 13.65,21.52 | 13.65,21.52 12.83,20.7 13.47,20.7 13.47,21.44 v13.62,21.59
  SUPPLY 0.813: 27.59,30.99 v27.59,30.1 27.59,26.95 26.55,25.91 16.26,25.91 13.62,23.27 v13.62,21.59 | 27.59,30.99 27.59,31.62 | 27.59,31.62 27.59,32 | v24.67,31.5 27.08,31.5 | 27.08,31.5 27.46,31.5 27.59,31.62 | 27.08,31.5 27.59,32 | 27.08,31.5 27.59,30.99 | 27.59,32 27.59,35.69 v28.86,36.96
  Bottom 0.305: A3V3.T 21.59,3.17 21.59,13.61 21.21,13.99 21.16,14.05 v13.62,21.59
AGND  (via drill 0.3 pad 0.64)
  Top 0.254: C19.1 26.06,36.2 | 26.06,36.2 27.59,36.2 | 26.06,36.2 6.63,36.2 4.7,34.27 4.7,28.7 5.2,28.21 J3.2 | U2.37 31.88,35.26 31.88,34.8 | U2.47 31.88,30.26 31.88,30.86 | U2.40 32.01,33.76 32.01,33.53 v32.03,33.53 32.03,33.26 U2.41 | C21.1 26.06,28.09 26.04,28.07 | 26.04,28.07 28.07,28.07 28.58,28.57 | 26.04,28.07 24.52,28.07
  Top 0.406: C20.1 24.77,33.02 | 24.77,33.02 C6.1 24.52,33.02 24.52,32.77 | C12.1 26.06,30.35 | 26.06,30.35 C21.1 | 18.35,31.88 23.63,31.88 24.77,33.02 | 18.16,30.36 18.17,30.35 | 18.17,30.35 15.12,30.35 14.89,30.58 D4.1 | 18.17,30.35 26.06,30.35 | 18.3,25.7 C22.1 | D3.1 14.89,24.64 15.27,24.26 26.17,24.26 30.45,28.54 v30.45,28.96 | C8.2 28.01,23.81 26.93,22.73 17.4,22.73 C35.1
  Top 1.016: v31.97,35.05 32.01,35.05 32.01,33.53 32.01,31.56 | 31.82,35.05 31.82,31.56
  other vias: 32.03,31.75 32.03,29.97 30.51,35.94 1.27,36.83 28.61,23.24 3.18,36.83 1.27,34.92 3.18,34.92 5.08,36.83 18.42,31.11 22.23,31.11 23.5,29.84 22.23,29.84 18.42,29.84 13.34,30.48 13.34,32.38 13.34,34.29 11.43,34.29 11.43,32.38 24.77,29.84 23.5,24.77 21.59,24.77 19.69,24.77 13.34,26.67 13.34,24.77 25.4,24.77 0.89,23.62 0.89,20.45 0.89,18.54 0.89,16.64 1.27,14.61 1.27,12.7 5.08,12.7 6.99,12.7 8.89,12.7 10.8,12.7 6.99,14.61 10.8,14.61 10.8,16.51 6.1,23.62 17.15,22.23 19.05,22.23 19.05,20.32 19.05,14.61 19.05,10.79 10.8,10.79 8.89,10.79 6.99,10.79 5.08,10.79 3.18,10.79 1.27,10.79 1.27,8.89 3.18,8.89 5.08,8.89 8.89,8.89 10.8,8.89 3.18,12.7 5.08,14.61 3.18,14.61 8.89,14.61 23.5,31.11 17.15,20.32 9.53,36.83 11.43,36.83 13.34,36.83 18.42,36.83 20.96,36.83 22.23,36.83 19.69,29.84 19.69,31.11 20.96,31.11 20.96,29.84 16.39,17.78 16.51,13.97 9.53,34.29 7.62,20.32
  pour Top (isolate 0.254): 0,8.26 19.69,8.26 19.69,22.23 32.39,22.23 32.39,37.47 0,37.47
  pour Bottom (isolate 0.254): 0,8.26 19.69,8.26 19.69,22.23 32.39,22.23 32.39,37.47 0,37.47
  pour GROUND (isolate 0.254): 0,8.26 19.69,8.26 19.69,22.23 32.39,22.23 32.39,37.47 0,37.47
GND  (via drill 0.3 pad 0.64)
  Top 0.152: v1.27,38.73 1.27,38.05 8.18,38.05 8.18,38.53
  Top 0.203: v1.27,38.73
  Top 0.254: 42.55,34.26 42.57,34.29 42.32,34.54 40.67,34.54 40.39,34.26 U2.22 38.08,34.26 37.98,34.16 37.98,33.78 | 42.57,29.72 41.94,30.35 40.42,30.35 40.03,30.73 40.03,31.11 39.89,31.26 U2.16 38,31.26 37.98,31.24 | U2.35 32.55,36.16 33.02,35.69 37.98,35.69 38.11,35.81 | U2.4 33.55,29.61 33.66,29.72 37.98,29.72 37.98,31.24 | 37.98,31.24 37.98,33.27 | 37.98,33.27 37.98,33.78 | U2.21 38,33.76 37.98,33.78 | U2.20 37.99,33.26 37.98,33.27 | U3.10 57.3,27.93 57.28,27.94 v56.51,27.94 | 0.47,39.67 0.47,46.19 D1.-
  Top 0.305: C13.1 41.03,27.94 41.53,27.43 43.06,27.43 43.82,28.19 | U3.1 55.91,30.57 v56.01,30.48 56.61,29.88 U3.13
  Top 0.406: U7.10 41.39,14.62 v41.4,14.61 | U7.7 44.35,15.97 v44.26,15.88 | U7.4 44.99,13.97 44.86,13.84 | U7.13 41.4,12.67 41.56,12.51 | C17.1 32.49,22.25 32.9,21.84 34.04,21.84 34.29,21.59
  Top 0.61: v34.8,33.53 32.01,33.53
  Top 0.813: v38.48,28.26 38.29,28.45 38.29,29.02 v37.34,29.97 | v37.34,35.05 38.11,35.81 38.42,36.12 38.42,37.24 39.4,38.23 | 39.5,38.23 40.51,38.23 C15.1
  other vias: 44.45,39.62 46.35,39.62 43.56,35.56 44.45,27.94 34.29,42.55 36.2,42.55 44.89,13.84 47.5,11.05 54.17,41.27 54.1,36.58 41.53,12.51 34.24,21.64 34.8,35.05 38.42,36.39 42.55,39.62 41.53,18.92 43.94,18.92 36.58,18.92 39.12,18.92 44.45,26.16 41.91,26.16 37.34,33.53 37.34,31.75 34.8,29.97 28.32,19.56 32.38,19.56 28.32,17.78 32.38,18.03 25.27,19.56 32.38,14.22 52.71,8.26 52.71,12.7 34.92,10.16 20.95,20.32 33.22,21.64 20.95,16.51 1.27,6.99 3.17,6.99 5.08,6.99 8.89,6.99 10.8,6.99 1.27,1.91 3.17,1.91 5.08,1.91 6.99,1.91 8.89,1.91 10.8,1.91 10.8,4.45 8.89,4.45 6.99,4.45 5.08,4.45 3.17,4.45 1.27,4.45 12.7,6.99 14.61,6.99 16.51,6.99 18.41,6.99 12.7,4.45 14.61,4.45 16.51,4.45 18.41,4.45 18.41,1.91 16.51,1.91 14.61,1.91 12.7,1.91 1.27,48.26 27.94,39.37 29.21,39.37 54.17,43.18 52.72,28.5 34.8,31.75 25.4,1.91 25.4,4.45 25.4,6.99 46.35,18.92 49.54,21.01 52.72,26.34 21.59,43.81 27.94,42.16 46.35,27.94 43.81,32 46.35,32 48.91,22.91 26.68,14.02 25.41,15.93 28.59,11.35 36.59,11.99 26.67,43.18
  pour Top (isolate 0.254): 0,7.62 20.32,7.62 20.32,21.59 33.02,21.59 33.02,38.1 0,38.1 0,53.34 68.58,53.34 68.58,0 0,0
  pour Bottom (isolate 0.254): 0,7.62 20.32,7.62 20.32,21.59 33.02,21.59 33.02,38.1 0,38.1 0,53.34 68.58,53.34 68.58,0 0,0
  pour GROUND (isolate 0.254): 0,7.62 20.32,7.62 20.32,21.59 33.02,21.59 33.02,38.1 0,38.1 0,53.34 68.58,53.34 68.58,0 0,0
GPIO0
  Top 0.254: U2.33 33.55,38.21 33.27,38.48 33.27,39.98 33.3,40.01 R6.2
GPIO1  (via drill 0.3 pad 0.64)
  Top 0.152: GPIO1.MM GPIO1.00
  Top 0.254: v47.62,39.5 48.89,38.23 48.89,26.16 46.61,23.88 46.61,22.86 | U2.34 33.05,38.1 32.54,38.61 32.54,43.02 32.96,43.43 v47.62,43.43 47.65,43.43
  Top 0.406: GPIO1.MM 46.61,22.86 | GPIO1.00 47.88,19.49 R15.1
  Bottom 0.254: v47.62,43.43 v47.62,39.5
GPIO2
  Top 0.152: GPIO2.MM GPIO2.00
  Top 0.254: U2.9 36.05,27.1 38.76,24.38 38.76,23.83 39.22,23.37 41.69,23.37 42.16,22.89 42.16,22.32
  Top 0.406: GPIO2.MM 42.16,22.32 | GPIO2.00 43.43,19.81 R17.1
GPIO3  (via drill 0.3 pad 0.64)
  Top 0.152: GPIO3.MM GPIO3.00
  Top 0.254: U2.10 36.55,27.35 38.73,25.17 38.74,25.17 39.56,24.35 v39.56,24.07
  Top 0.406: GPIO3.MM 37.72,22.14 38.18,22.61 v38.73,22.61 | GPIO3.00 38.99,20.26 R19.1
  Bottom 0.254: v39.56,24.07 38.73,23.24 v38.73,22.61
I2S_DATA  (via drill 0.3 pad 0.64)
  Top 0.254: U2.12 37.55,27.86 40.77,24.64 45.88,24.64 47.88,26.64 47.88,37.21 v47.62,37.47 | R12.2 60.96,37.47 J1.4
  Bottom 0.254: v47.62,37.47 60.96,37.47 J1.4
I2S_LROUT
  Top 0.254: U2.36 32.05,43.8 32.03,43.81 33.18,44.96 55.02,44.96 | 55.47,44.96 60.83,44.96 J1.1 | 55.47,44.96 55.15,44.96 | 55.15,44.96 55.02,44.96 | R8.2 55.24,44.73 | 55.24,44.74 55.24,44.86 55.15,44.96 | 55.24,44.73 55.02,44.96 | 55.24,44.73 55.24,44.74 | 55.24,44.74 55.47,44.96
I2S_MCLK  (via drill 0.3 pad 0.64)
  Top 0.254: U2.25 37.55,37.67 40.51,40.64 48.13,40.64 v48.77,40.01 | 59.56,41.27 R9.2 59.69,41.27 J1.2
  Bottom 0.254: v48.77,40.01 58.42,40.01 J1.2
I2S_SCLK  (via drill 0.3 pad 0.64)
  Top 0.254: U2.11 37.05,27.59 40.51,24.13 46.13,24.13 48.39,26.39 48.39,37.72 v47.62,38.48 | R11.2 60.32,39.37 J1.3
  Bottom 0.254: v47.62,38.48 59.44,38.48 J1.3
K_BK  (via drill 0.3 pad 0.64)
  Top 0.305: U10.7 48.26,48.39 47.38,47.5 29.34,47.5 v29.21,47.62 | v29.21,44.7 C39.1 | v11.82,42.16 9.87,42.16 K1.2
  Bottom 0.305: v11.82,42.16 26.67,42.16 v29.21,44.7 v29.21,47.62
K_NT
  Top 0.305: U10.5 53.34,46.86 52.71,46.23 24.39,46.23 23.75,45.59 23.75,41.88 C41.1 21.85,41.02 20.77,42.09 K1.5
K_PS
  Top 0.305: U10.6 50.8,47.62 50.04,46.86 23.37,46.86 22.89,46.38 C42.1 22.1,44.7 21.01,45.8 K1.6
K_VD  (via drill 0.3 pad 0.64)
  Top 0.305: U10.8 45.72,48.9 44.94,48.11 30.64,48.11 v30.48,48.26 | C38.1 v27.69,41.02 | v11.82,39.37 9.87,39.37 K1.3
  Bottom 0.305: v30.48,48.26 30.48,43.81 v27.69,41.02 26.04,39.37 v11.82,39.37
K_VU  (via drill 0.3 pad 0.64)
  Top 0.305: U10.4 55.88,47.5 53.98,45.59 26.32,45.59 C40.1 25.4,44.7 25.15,44.96 v24.52,44.96 | 10.16,45.85 10.17,45.84 9.87,45.84 K1.1 9.87,45.85 v11.82,45.85
  Bottom 0.305: v11.82,45.85 12.7,44.96 v24.52,44.96
LEFT
  Top 0.406: C1.- 18.38,28.49 18.17,28.7 R22.2 16.56,28.81 D3.2 11.7,28.81 8.64,31.88 8.64,32.24 J3.4 8.26,32.55
MIC
  Top 0.406: R7.2 5.71,19.18 C11.2 5.46,22.48 C10.1 1.95,22.48 D2.2 2,22.53 J3.1
MIDI_IN
  Top 0.254: R3.2 61.59,35.56 J1.5
MISO  (via drill 0.3 pad 0.64)
  Top 0.254: U2.30 35.05,38.19 39.53,42.67 49.56,42.67 51.59,40.64 51.59,34.29 v51.21,33.91 | U3.12 57.52,29.21 v55.91,29.21 55.35,29.21 54.89,28.75 54.89,16.76 arc-90 54.64,16.51 53.05,16.51 arc90 52.8,16.26 arc90 53.05,16 54.64,16 arc-90 54.89,15.75 arc-90 54.64,15.49 53.05,15.49 arc90 52.8,15.24 arc90 53.05,14.99 54.64,14.99 arc-90 54.89,14.73 arc-90 54.64,14.48 53.05,14.48 arc90 52.8,14.22 arc90 53.05,13.97 54.64,13.97 arc-90 54.89,13.72 54.89,12.09 54.33,11.53 U5.7
  Bottom 0.254: v51.21,33.91 51.21,33.81 55.81,29.21 v55.91,29.21
MISO_A  (via drill 0.3 pad 0.64)
  Top 0.254: U10.38 62.23,29.21 v62.23,24.13
  Bottom 0.254: v62.23,24.13 MISO.00 59.06,24.13
MISO_B
  Bottom 0.254: MISO.11 50.8,24.13 50.55,24.38
  Bottom 0.305: 50.68,24.26 50.55,24.38 49.53,25.4 49.53,27.56 47.63,29.46 47.63,35.31 44.84,38.1 34.73,38.1 31.75,41.08 31.75,50.55 U10.13
MOSI  (via drill 0.3 pad 0.64)
  Top 0.254: U2.29 35.55,37.93 39.78,42.16 49.31,42.16 51.08,40.39 51.08,34.92 50.45,34.29 50.45,33.66 v49.69,32.89 | U3.6 52.83,27.27 v52.86,27.3 53.62,27.3 53.88,27.05 53.88,25.81 53.59,25.53 52.61,25.53 arc90 52.35,25.27 arc90 52.61,25.02 53.62,25.02 arc-90 53.88,24.77 arc-90 53.62,24.51 52.61,24.51 arc90 52.35,24.26 arc90 52.61,24 53.62,24 arc-90 53.88,23.75 arc-90 53.62,23.5 52.61,23.5 arc90 52.35,23.24 arc90 52.61,22.99 53.62,22.99 arc-90 53.88,22.73 arc-90 53.62,22.48 52.61,22.48 arc90 52.35,22.23 arc90 52.61,21.97 53.62,21.97 arc-90 53.88,21.72 arc-90 53.62,21.46 52.59,21.46 arc45 52.41,21.39 arc90 52.41,21.03 arc45 52.59,20.95 53.62,20.95 arc-90 53.88,20.7 arc-90 53.62,20.45 52.61,20.45 arc90 52.35,20.19 arc90 52.61,19.94 53.62,19.94 arc-90 53.88,19.68 arc-90 53.62,19.43 49.03,19.43 48.67,19.07 48.67,16.23 48.98,15.93 U5.3
  Bottom 0.254: v49.69,32.89 49.87,32.89 53.46,29.3 53.46,27.9 v52.86,27.3 52.84,27.3
MOSI_A
  Bottom 0.254: U10.34 64.77,26.67 MOSI.11 59.06,26.67
MOSI_B
  Bottom 0.254: 45.22,38.73 34.93,38.73 32.39,41.27 32.39,49.15 U10.12
  Bottom 0.305: MOSI.00 56.52,25.4 50.8,25.4 50.17,26.04 50.17,27.94 48.26,29.84 48.26,35.69 45.22,38.73
MSD_CS  (via drill 0.3 pad 0.64)
  Top 0.254: v36.58,44.2 48.8,44.2 52.23,40.77 52.23,32.13 51.46,31.37 R26.1
  Bottom 0.254: v36.58,44.2 U10.11
N$1
  Top 0.254: X1.2 43.69,32.77 C5.2 R5.1 40.92,32.77 40.42,32.26 U2.18
N$2
  Top 0.254: X1.1 43.69,31.24 C7.2 R5.2 40.44,31.76 U2.17
N$3
  Top 0.254: U2.44 28.11,31.76 C12.2
N$4
  Top 0.406: R10.2 7.49,17.53 R7.1 5.27,17.53 C30.+
N$5
  Top 0.406: C22.2 R22.1
N$6
  Top 0.254: U2.39 29.58,34.26 arc-45 29.26,34.4 28.86,34.8
  Top 0.406: 28.86,34.8 28.32,35.33 arc45 27.77,35.56 23.94,35.56 arc45 C37.1 21.72,35.18 21.39,34.84 C2.+
N$7
  Top 0.254: U2.2 32.55,27.44 32.16,27.05 31.53,27.05 29.84,25.37 C8.1 29.84,25.3
N$8
  Top 0.254: U2.46 29.69,30.76 arc90 29.37,30.44 29.37,30.23
  Top 0.406: 29.37,29.19 29.37,29.21 | 29.37,29.21 29.37,30.23 | 29.37,29.21 arc-90 27.46,27.3 25.38,27.3 arc-45 23.69,28.01 C31.1 | C31.1 21.72,28.7 21.3,28.28 C1.+ | C31.1
N$9
  Top 0.406: C6.2 R4.2
N$10
  Top 0.406: R21.1 16.79,32.09 C23.2
N$11
  Top 0.254: U2.1 31.53,28.26
  Top 0.406: 31.97,28.26 31.53,28.26 31.08,28.26 26.19,23.37 10.42,23.37 9.15,22.1 7.62,22.1 C11.1 7.49,22.45
N$12  (via drill 0.3 pad 0.64)
  Top 0.254: U2.26 37.05,37.94 40.26,41.15 48.77,41.15 49.66,40.26 v49.66,35.69 | R2.2 R3.1 v54.1,35.56
  Bottom 0.254: v49.66,35.69 54,35.69 54.13,35.56 v54.1,35.56
N$13
  Top 0.813: U1.3 24.81,11.49 C3.2 27.05,9.43 | U6.3 30.52,11.49 C24.2 32.77,9.53 C29.+ 32.16,8.91 | 27.18,8.91 32.16,8.91 | U8.3 14.39,11.18 14.38,11.18 14.63,11.43 C32.2 19.47,8.91 27.18,8.91 | 27.05,9.37 27.05,9.05 27.18,8.91 | 27.05,9.43 27.05,9.37 | 27.05,9.37 26.7,9.02 | 27.05,9.43 27.46,9.02 | L2.2 36.83,8.63 35.69,7.49 33.41,7.49 32.26,8.64 32.26,8.81 32.16,8.91
N$14
  Top 0.254: R31.2 41.43,6.6 43.97,4.06 49.28,4.06 U10.19
N$15
  Top 0.254: U2.42 29.37,32.76 R4.1
N$16
  Top 0.254: U3.2 49.97,29.88 R26.2
N$17
  Top 0.254: U7.2 45.34,12.67 44.99,12.32 44.99,10.67 45.5,10.16 R29.1
  pour Top (no thermals): 2.34,41.91 2.84,42.37 2.84,41.45
  pour Top (no thermals): 1.68,41.91 2.19,42.37 2.19,41.45
N$18
  Top 0.254: U3.5 50.21,27.93 R27.2
N$19
  Top 0.254: R30.1 43.97,14.1 44.48,14.61 46.09,14.61 U7.5
N$20
  Top 0.254: U7.12 42.05,13.32 42.38,12.99 42.38,11.11 R31.1
N$21
  Top 0.254: U3.3 53.86,29.23 54.39,28.7 54.39,17.73 53.68,17.02 U5.2
N$22
  Top 0.254: R29.2 46.51,7.19 47.99,5.71 55.25,5.71 U10.22
N$23
  Top 0.254: R30.2 43.97,7.24 46,5.21 53.22,5.21 U10.21
  pour Top (no thermals): 6.71,42.37 6.71,41.45 7.21,41.91
N$24
  Top 0.254: U7.8 41.97,15.97 42.96,14.99 42.96,6.99 45.25,4.7 51.19,4.7 U10.20
N$25
  pour Top (no thermals): 3.89,42.37 4.42,41.91 3.89,41.45
N$27
  pour Top (no thermals): 6.71,42.37 7.21,41.91 6.71,41.45
N$28
  pour Top (no thermals): 6.05,42.37 6.05,41.45 6.55,41.91
N$29
  Top 0.152: 5.05,42.37 5.05,41.45
N$30
  Top 0.152: 3.81,43.94 3.49,43.94 3.49,44.45 3.81,44.45 | 3.81,43.94 3.81,44.45 | 3.81,44.45 4.32,44.83 arc-19 4.32,43.56 3.81,43.94
N$31
  Top 0.152: 4.7,44.2 5.33,44.2
N$32
  Top 0.152: 5.02,44.51 5.02,43.88
N$34
  Top 0.152: 3.81,39.37 3.49,39.37 3.49,39.88 3.81,39.88 | 3.81,39.37 3.81,39.88 | 3.81,39.88 4.32,40.26 arc-19 4.32,38.99 3.81,39.37
N$35
  Top 0.152: 4.7,39.62 5.33,39.62
N$36
  Top 0.305: U3.11 58.99,28.57 R23.2 R20.1
N$37
  Top 0.254: D1.+ R13.1
N$38
  Top 0.254: U7.9 38.73,15.27 38.03,15.97 R25.1
N$39  (via drill 0.3 pad 0.64)
  Top 0.254: R20.2 60.96,30.35 61.73,29.59 61.73,25.53 v61.6,25.4
  Bottom 0.254: v61.6,25.4 59.44,25.4 59.06,25.02 MISO.MM
N$40
  Top 0.406: U3.9 58.99,27.27 R28.2
N$41
  Top 0.152: 1.4,42.37 1.4,41.45
  pour Top (isolate 0.254, no thermals): 2.19,42.37 2.19,41.45 1.68,41.91
N$42
  pour Top (isolate 0.254, no thermals): 2.34,41.91 2.84,42.37 2.84,41.45 2.34,41.91
N$43
  Top 0.152: 4.75,42.37 4.75,41.45
N$44
  pour Top: 1.68,41.92 2.19,42.37 2.19,41.45 1.68,41.91
N$45
  Top 0.152: 7.5,42.37 7.5,41.45
N$49  (via drill 0.3 pad 0.64)
  Top 0.254: v51.44,24.77 50.8,24.77 49.94,25.63 R27.1
  Bottom 0.254: MOSI.MM 59.06,25.91 58.55,25.4 57.28,25.4 56.65,24.77 v51.44,24.77
N$53  (via drill 0.3 pad 0.64)
  Top 0.254: R28.1 60.71,27.05 58.42,24.77 v58.42,22.86
  Bottom 0.254: v58.42,22.86 59.06,22.23 SCK.MM
PULL_UP1
  Top 0.406: GPIO1.11 45.34,19.3 R14.1
PULL_UP2
  Top 0.406: GPIO2.11 40.89,19.68 R16.1
PULL_UP3
  Top 0.406: GPIO3.11 36.45,20.19 R18.1
RIGHT
  Top 0.203: 6.06,32.65 6,32.65 J3.7
  Top 0.406: C2.- 18.47,35.13 18.42,35.18 R21.2 14.9,35.18 D4.2 6.98,35.16 arc90 6.06,34.24 6.06,32.65 | J3.7 6,30.07 7.75,28.32 7.75,25.98 J3.3
SCK  (via drill 0.3 pad 0.64)
  Top 0.254: U2.28 36.05,37.67 40.03,41.66 49.05,41.66 50.58,40.13 50.58,35.43 49.69,34.54 v49.69,34.16 | U3.8 56.07,26.57 v55.53,26.04 55.53,7.64 54.61,6.73 49.15,6.73 48.26,7.62 48.26,13.21 48.78,13.72 U5.5
  Bottom 0.254: v55.53,26.04 55.53,28.32 v49.69,34.16
SCK_A  (via drill 0.3 pad 0.64)
  Top 0.254: U10.37 64.77,26.67 64.77,22.86 63.5,21.59 v61.6,21.59
  Bottom 0.254: v61.6,21.59 SCK.11 59.06,21.59
SCK_B
  Bottom 0.305: U10.14 31.12,48.64 31.12,40.79 34.44,37.47 44.45,37.47 46.99,34.92 46.99,29.21 48.9,27.3 48.9,25.15 50.55,23.5 55.88,23.5 SCK.00
VOLUME
  Top 0.305: U10.9 40.14,49.28 19.82,49.28 18.17,47.62 11.94,47.62 10.93,48.64 R13.2
VS_DREQ
  Top 0.254: U2.8 35.55,26.97 37.49,25.02 37.49,23.62 34.45,20.57 34.45,14.73 34.83,14.35 R24.2 R25.2
VS_XCS  (via drill 0.3 pad 0.64)
  Top 0.254: U2.23 40.1,34.76 41.66,36.32 46.64,36.32 47.4,35.56 47.4,27.08 v46.99,26.67 | U7.3 46.97,13.32 v46.99,13.34
  Bottom 0.254: v46.99,13.34 47.63,13.97 47.63,26.03 v46.99,26.67
VS_XDCS  (via drill 0.3 pad 0.64)
  Top 0.254: U2.13 39.48,29.76 39.91,29.34 39.91,27.56 40.54,26.92 45.88,26.92 v46.13,26.67 | U7.6 46.99,15.27 v47.02,15.24
  Bottom 0.254: v47.02,15.24 47.02,25.78 v46.13,26.67
VS_XRESET
  Top 0.254: U7.11 39.37,13.97 R1.1 38.1,12.73 37.3,13.53 34.64,13.53 33.94,14.22 33.94,19.71 30.74,22.91 30.74,25.43 31.85,26.54 32.41,26.54 33.05,27.18 U2.3
(copper drawn outside any net)
  shapes: Top circle x1

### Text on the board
tPlace: SCL | 13 | 12 | 11 | 10 | 9 | 8 | 7 | 6 | 5 | 4 | 3 | 2 | 1 | 0 | SDA | GND | AREF | DIGITAL | LROUT | MCLK | I2S | SCLK | DATA | MIDI | GND | H | L | H | L | H | L | ANALOG | NC | IOREF | RST | 3V3 | 5V | GND | GND | VIN | 0 | 1 | 2 | 3 | 4 | 5
bPlace: Music Shield | B | A | v2.2 11/28/2014 | B | A | by Seeed Studio | B | A | www.seeedstudio.com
